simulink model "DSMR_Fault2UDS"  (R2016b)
settings: Solver=FixedStepDiscrete  StartTime=0.0  StopTime=10.0  FixedStep=0.02  RelTol=1e-3  EnableMultiTasking=on
undefined symbols (not defined in the file): bin2dec
libraries: simulink x312
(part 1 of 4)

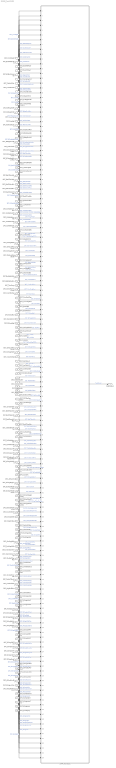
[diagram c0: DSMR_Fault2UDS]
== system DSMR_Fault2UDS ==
  DFC_CurrRngErr : Inport
  DFC_BattVoltRngErr : Inport  Port=2
  DFC_BattHVMsgTmt : Inport  Port=3
  DFC_BusHVMsgTmt : Inport  Port=4
  DFC_638LinCommErr : Inport  Port=5
  DFC_CellTempTmt : Inport  Port=6
  DFC_CellVoltTmt : Inport  Port=7
  DFC_InCanBusOff : Inport  Port=8
  DFC_VeCanBusOff : Inport  Port=9
  DFC_Msg2A3Tmt : Inport  Port=10
  DFC_RcMsg2A3Mis : Inport  Port=11
  DFC_ChkSumMsg2A3Err : Inport  Port=12
  DFC_RcMsg2A5Mis : Inport  Port=13
  DFC_RcMsg2A7Mis : Inport  Port=14
  DFC_CrashNpl : Inport  Port=15
  DFC_FuseNpl : Inport  Port=16
  DFC_Kl30cVoltLoErr : Inport  Port=17
  DFC_PosStuckMax : Inport  Port=18
  DFC_MPosStuckMin : Inport  Port=19
  DFC_MNegStuckMax : Inport  Port=20
  DFC_MNegStuckMin : Inport  Port=21
  DFC_PrStuckMin : Inport  Port=22
  DFC_DChrgPosStuckMax : Inport  Port=23
  DFC_DChrgPosStuckMin : Inport  Port=24
  DFC_DChrgNegStuckMax : Inport  Port=25
  DFC_DChrgNegStuckMin : Inport  Port=26
  DFC_HvPwrUpFail : Inport  Port=27
  DFC_DChrgPwrUpFail : Inport  Port=28
  DFC_BattTAlrmMax : Inport  Port=29
  DFC_BattTFaultMax : Inport  Port=30
  DFC_BattTAlrmMin : Inport  Port=31
  DFC_BattTFaultMin : Inport  Port=32
  DFC_BattTempVldMin : Inport  Port=33
  DFC_BattTCnstMax : Inport  Port=34
  DFC_BattTGradtMax : Inport  Port=35
  DFC_CellVoltAlrmMax : Inport  Port=36
  DFC_CellVoltFaultMax : Inport  Port=37
  DFC_CellVoltFusfMax : Inport  Port=38
  DFC_CellVoltAlrmMin : Inport  Port=39
  DFC_CellVoltFusfMin : Inport  Port=40
  DFC_CellVoltFaultMin : Inport  Port=41
  DFC_CellVoltVldMin : Inport  Port=42
  DFC_CellVoltNpl : Inport  Port=43
  DFC_Msg2E6Tmt : Inport  Port=44
  DFC_RcMsg2E6Mis : Inport  Port=45
  DFC_ChkSumMsg2E6Err : Inport  Port=46
  DFC_RcMsg2E1Mis : Inport  Port=47
  DFC_ChkSumMsg2E1Err : Inport  Port=48
  DFC_DcCanBusOff : Inport  Port=49
  DFC_DChrgTCnntMax : Inport  Port=50
  DFC_ChrgOCNpl : Inport  Port=51
  DFC_DisChOCNpl : Inport  Port=52
  DFC_BattVoltHiMax : Inport  Port=53
  DFC_BattVoltLoMin : Inport  Port=54
  DFC_ThmRnwy : Inport  Port=55
  DFC_AChrgPortOvrTemp : Inport  Port=56
  DFC_CurrOffsPlaus : Inport  Port=57
  DFC_CurrStukPlaus : Inport  Port=58
  DFC_CurrChrgPlaus : Inport  Port=59
  DFC_BattUNpl : Inport  Port=60
  DFC_BattVoltVld : Inport  Port=61
  DFC_PackUNpl : Inport  Port=62
  DFC_PackVoltVld : Inport  Port=63
  DFC_DChrgUNpl : Inport  Port=64
  DFC_DChrgVoltVld : Inport  Port=65
  DFC_BoardTempTmt : Inport  Port=66
  DFC_HvilMax : Inport  Port=67
  DFC_HvilMin : Inport  Port=68
  DFC_HvilSig : Inport  Port=69
  DFC_ChkSumMsg050Err : Inport  Port=70
  DFC_RcMsg050Mis : Inport  Port=71
  DFC_CrashHwNpl : Inport  Port=72
  DFC_IsoChkLv1 : Inport  Port=73
  DFC_IsoChkLv2 : Inport  Port=74
  DFC_InsResValdFault : Inport  Port=75
  DFC_Kl30OutRngErr : Inport  Port=76
  DFC_Kl30VoltLoErr : Inport  Port=77
  DFC_Kl30VoltHiErr : Inport  Port=78
  DFC_EepReadErr : Inport  Port=79
  DFC_BalStuckMax : Inport  Port=80
  DFC_BalStuckMin : Inport  Port=81
  DFC_CSCPwrSpyHiErr : Inport  Port=82
  DFC_CSCPwrSpyLoErr : Inport  Port=83
  DFC_CmcBordOTMax : Inport  Port=84
  DFC_BattTWarnMax : Inport  Port=85
  DFC_BattTWarnMin : Inport  Port=86
  DFC_BattTempVldMax : Inport  Port=87
  DFC_BattTHopMax : Inport  Port=88
  DFC_CellVoltRngHiErr : Inport  Port=89
  DFC_CellVoltRngLoErr : Inport  Port=90
  DFC_CellVoltWarnMax : Inport  Port=91
  DFC_CellVoltWarnMin : Inport  Port=92
  DFC_CellVoltVldMax : Inport  Port=93
  DFC_AChrgCurrMish : Inport  Port=94
  DFC_DChrgCurrMish : Inport  Port=95
  DFC_DChrgLowTempCurrMish : Inport  Port=96
  DFC_AChrgVoltMish : Inport  Port=97
  DFC_DChrgVoltMish : Inport  Port=98
  DFC_DChrgBattTMin : Inport  Port=99
  DFC_CC2Chk : Inport  Port=100
  DFC_APlusChk : Inport  Port=101
  DFC_DChrgMsgTmt : Inport  Port=102
  DFC_DChrgTNegElecMax : Inport  Port=103
  DFC_DChrgTNegElecMin : Inport  Port=104
  DFC_DChrgTNegElecSig : Inport  Port=105
  DFC_DChrgTPosElecMax : Inport  Port=106
  DFC_DChrgTPosElecMin : Inport  Port=107
  DFC_DChrgTPosElecSig : Inport  Port=108
  DFC_CcuSelfChkErr : Inport  Port=109
  DFC_ChrgOCMin : Inport  Port=110
  DFC_ChrgOCMax : Inport  Port=111
  DFC_DisChOCMin : Inport  Port=112
  DFC_DisChOCMax : Inport  Port=113
  DFC_SocRngLoMax : Inport  Port=114
  DFC_SocRngLoMin : Inport  Port=115
  DFC_SocRngHiMax : Inport  Port=116
  DFC_SocRngHiMin : Inport  Port=117
  DFC_InClntOverTmp : Inport  Port=118
  DFC_OutClntOverTmp : Inport  Port=119
  DFC_ClntDsTElecMax : Inport  Port=120
  DFC_ClntDsTElecMin : Inport  Port=121
  DFC_ClntDsTElecSig : Inport  Port=122
  DFC_ClntUsTElecMax : Inport  Port=123
  DFC_ClntUsTElecMin : Inport  Port=124
  DFC_ClntUsTElecSig : Inport  Port=125
  DFC_CoolPerfPlaus : Inport  Port=126
  DFC_HtgPerfPlaus : Inport  Port=127
  DFC_DChrgFobd : Inport  Port=128
  DFC_DChrgHvOnFail : Inport  Port=129
  DFC_AChgHVOnTmt : Inport  Port=130
  DFC_AChgHVOffTmt : Inport  Port=131
  DFC_AChgS2ClsdTmt : Inport  Port=132
  DFC_DChrgStakeErr : Inport  Port=133
  DFC_DChrgStkVoltErr : Inport  Port=134
  DFC_DChrgStkCurrErr : Inport  Port=135
  DFC_AChgPileRdyTmt : Inport  Port=136
  DFC_DChrgCHMTmt : Inport  Port=137
  DFC_DChrgCRMTmt : Inport  Port=138
  DFC_DChrgCMLTmt : Inport  Port=139
  DFC_DChrgCROTmt : Inport  Port=140
  DFC_DChrgCCSTmt : Inport  Port=141
  DFC_DChrgCSTTmt : Inport  Port=142
  DFC_DChrgCSDTmt : Inport  Port=143
  DFC_DChrgParaChk : Inport  Port=144
  DFC_DChrgCableChk : Inport  Port=145
  DFC_DChrgSLACTOut : Inport  Port=146
  DFC_DChrgCnntErr : Inport  Port=147
  DFC_DChrgLckErr : Inport  Port=148
  DFC_AChrgCnntErr : Inport  Port=149
  DFC_AChgLckTmt : Inport  Port=150
  DFC_AChgRdyPndiTmt : Inport  Port=151
  DFC_AChgRdyTmt : Inport  Port=152
  DFC_AChgingErr : Inport  Port=153
  DFC_AChgUnlckTmt : Inport  Port=154
  DFC_AChgFobd : Inport  Port=155
  DFC_SocValJmp : Inport  Port=156
  DSMR_Fault2UDS : Subsystem
  FaultStatus : Outport
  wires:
  DFC_CurrRngErr/1 -> DSMR_Fault2UDS/1(DFC_CurrRngErr)  "DFC_CurrRngErr"
  DFC_BattVoltRngErr/1 -> DSMR_Fault2UDS/2(DFC_BattVoltRngErr)  "DFC_BattVoltRngErr"
  DFC_BattHVMsgTmt/1 -> DSMR_Fault2UDS/3(DFC_BattHVMsgTmt)  "DFC_BattHVMsgTmt"
  DFC_BusHVMsgTmt/1 -> DSMR_Fault2UDS/4(DFC_BusHVMsgTmt)  "DFC_BusHVMsgTmt"
  DFC_638LinCommErr/1 -> DSMR_Fault2UDS/5(DFC_638LinCommErr)  "DFC_638LinCommErr"
  DFC_CellTempTmt/1 -> DSMR_Fault2UDS/6(DFC_CellTempTmt)  "DFC_CellTempTmt"
  DFC_CellVoltTmt/1 -> DSMR_Fault2UDS/7(DFC_CellVoltTmt)  "DFC_CellVoltTmt"
  DFC_InCanBusOff/1 -> DSMR_Fault2UDS/8(DFC_InCanBusOff)  "DFC_InCanBusOff"
  DFC_VeCanBusOff/1 -> DSMR_Fault2UDS/9(DFC_VeCanBusOff)  "DFC_VeCanBusOff"
  DFC_Msg2A3Tmt/1 -> DSMR_Fault2UDS/10(DFC_Msg2A3Tmt)  "DFC_Msg2A3Tmt"
  DFC_RcMsg2A3Mis/1 -> DSMR_Fault2UDS/11(DFC_RcMsg2A3Mis)  "DFC_RcMsg2A3Mis"
  DFC_ChkSumMsg2A3Err/1 -> DSMR_Fault2UDS/12(DFC_ChkSumMsg2A3Err)  "DFC_ChkSumMsg2A3Err"
  DFC_RcMsg2A5Mis/1 -> DSMR_Fault2UDS/13(DFC_RcMsg2A5Mis)  "DFC_RcMsg2A5Mis"
  DFC_RcMsg2A7Mis/1 -> DSMR_Fault2UDS/14(DFC_RcMsg2A7Mis)  "DFC_RcMsg2A7Mis"
  DFC_CrashNpl/1 -> DSMR_Fault2UDS/15(DFC_CrashNpl)  "DFC_CrashNpl"
  DFC_FuseNpl/1 -> DSMR_Fault2UDS/16(DFC_FuseNpl)  "DFC_FuseNpl"
  DFC_Kl30cVoltLoErr/1 -> DSMR_Fault2UDS/17(DFC_Kl30cVoltLoErr)  "DFC_Kl30cVoltLoErr"
  DFC_PosStuckMax/1 -> DSMR_Fault2UDS/18(DFC_PosStuckMax)  "DFC_PosStuckMax"
  DFC_MPosStuckMin/1 -> DSMR_Fault2UDS/19(DFC_MPosStuckMin)  "DFC_MPosStuckMin"
  DFC_MNegStuckMax/1 -> DSMR_Fault2UDS/20(DFC_MNegStuckMax)  "DFC_MNegStuckMax"
  DFC_MNegStuckMin/1 -> DSMR_Fault2UDS/21(DFC_MNegStuckMin)  "DFC_MNegStuckMin"
  DFC_PrStuckMin/1 -> DSMR_Fault2UDS/22(DFC_PrStuckMin)  "DFC_PrStuckMin"
  DFC_DChrgPosStuckMax/1 -> DSMR_Fault2UDS/23(DFC_DChrgPosStuckMax)  "DFC_DChrgPosStuckMax"
  DFC_DChrgPosStuckMin/1 -> DSMR_Fault2UDS/24(DFC_DChrgPosStuckMin)  "DFC_DChrgPosStuckMin"
  DFC_DChrgNegStuckMax/1 -> DSMR_Fault2UDS/25(DFC_DChrgNegStuckMax)  "DFC_DChrgNegStuckMax"
  DFC_DChrgNegStuckMin/1 -> DSMR_Fault2UDS/26(DFC_DChrgNegStuckMin)  "DFC_DChrgNegStuckMin"
  DFC_HvPwrUpFail/1 -> DSMR_Fault2UDS/27(DFC_HvPwrUpFail)  "DFC_HvPwrUpFail"
  DFC_DChrgPwrUpFail/1 -> DSMR_Fault2UDS/28(DFC_DChrgPwrUpFail)  "DFC_DChrgPwrUpFail"
  DFC_BattTAlrmMax/1 -> DSMR_Fault2UDS/29(DFC_BattTAlrmMax)  "DFC_BattTAlrmMax"
  DFC_BattTFaultMax/1 -> DSMR_Fault2UDS/30(DFC_BattTFaultMax)  "DFC_BattTFaultMax"
  DFC_BattTAlrmMin/1 -> DSMR_Fault2UDS/31(DFC_BattTAlrmMin)  "DFC_BattTAlrmMin"
  DFC_BattTFaultMin/1 -> DSMR_Fault2UDS/32(DFC_BattTFaultMin)  "DFC_BattTFaultMin"
  DFC_BattTempVldMin/1 -> DSMR_Fault2UDS/33(DFC_BattTempVldMin)  "DFC_BattTempVldMin"
  DFC_BattTCnstMax/1 -> DSMR_Fault2UDS/34(DFC_BattTCnstMax)  "DFC_BattTCnstMax"
  DFC_BattTGradtMax/1 -> DSMR_Fault2UDS/35(DFC_BattTGradtMax)  "DFC_BattTGradtMax"
  DFC_CellVoltAlrmMax/1 -> DSMR_Fault2UDS/36(DFC_CellVoltAlrmMax)  "DFC_CellVoltAlrmMax"
  DFC_CellVoltFaultMax/1 -> DSMR_Fault2UDS/37(DFC_CellVoltFaultMax)  "DFC_CellVoltFaultMax"
  DFC_CellVoltFusfMax/1 -> DSMR_Fault2UDS/38(DFC_CellVoltFusfMax)  "DFC_CellVoltFusfMax"
  DFC_CellVoltAlrmMin/1 -> DSMR_Fault2UDS/39(DFC_CellVoltAlrmMin)  "DFC_CellVoltAlrmMin"
  DFC_CellVoltFusfMin/1 -> DSMR_Fault2UDS/40(DFC_CellVoltFusfMin)  "DFC_CellVoltFusfMin"
  DFC_CellVoltFaultMin/1 -> DSMR_Fault2UDS/41(DFC_CellVoltFaultMin)  "DFC_CellVoltFaultMin"
  DFC_CellVoltVldMin/1 -> DSMR_Fault2UDS/42(DFC_CellVoltVldMin)  "DFC_CellVoltVldMin"
  DFC_CellVoltNpl/1 -> DSMR_Fault2UDS/43(DFC_CellVoltNpl)  "DFC_CellVoltNpl"
  DFC_Msg2E6Tmt/1 -> DSMR_Fault2UDS/44(DFC_Msg2E6Tmt)  "DFC_Msg2E6Tmt"
  DFC_RcMsg2E6Mis/1 -> DSMR_Fault2UDS/45(DFC_RcMsg2E6Mis)  "DFC_RcMsg2E0Mis"
  DFC_ChkSumMsg2E6Err/1 -> DSMR_Fault2UDS/46(DFC_ChkSumMsg2E6Err)  "DFC_ChkSumMsg2E0Err"
  DFC_RcMsg2E1Mis/1 -> DSMR_Fault2UDS/47(DFC_RcMsg2E1Mis)  "DFC_RcMsg2E1Mis"
  DFC_ChkSumMsg2E1Err/1 -> DSMR_Fault2UDS/48(DFC_ChkSumMsg2E1Err)  "DFC_ChkSumMsg2E1Err"
  DFC_DcCanBusOff/1 -> DSMR_Fault2UDS/49(DFC_DcCanBusOff)  "DFC_DcCanBusOff"
  DFC_DChrgTCnntMax/1 -> DSMR_Fault2UDS/50(DFC_DChrgTCnntMax)  "DFC_DChrgTCnntMax"
  DFC_ChrgOCNpl/1 -> DSMR_Fault2UDS/51(DFC_ChrgOCNpl)  "DFC_ChrgOCNpl"
  DFC_DisChOCNpl/1 -> DSMR_Fault2UDS/52(DFC_DisChOCNpl)  "DFC_DisChOCNpl"
  DFC_BattVoltHiMax/1 -> DSMR_Fault2UDS/53(DFC_BattVoltHiMax)  "DFC_BattVoltHiMax"
  DFC_BattVoltLoMin/1 -> DSMR_Fault2UDS/54(DFC_BattVoltLoMin)  "DFC_BattVoltLoMin"
  DFC_ThmRnwy/1 -> DSMR_Fault2UDS/55(DFC_ThmRnwy)  "DFC_ThmRnwy"
  DFC_AChrgPortOvrTemp/1 -> DSMR_Fault2UDS/56(DFC_AChrgPortOvrTemp)  "DFC_AChrgPortOvrTemp"
  DFC_CurrOffsPlaus/1 -> DSMR_Fault2UDS/57(DFC_CurrOffsPlaus)  "DFC_CurrOffsPlaus"
  DFC_CurrStukPlaus/1 -> DSMR_Fault2UDS/58(DFC_CurrStukPlaus)  "DFC_CurrStukPlaus"
  DFC_CurrChrgPlaus/1 -> DSMR_Fault2UDS/59(DFC_CurrChrgPlaus)  "DFC_CurrChrgPlaus"
  DFC_BattUNpl/1 -> DSMR_Fault2UDS/60(DFC_BattUNpl)  "DFC_BattUNpl"
  DFC_BattVoltVld/1 -> DSMR_Fault2UDS/61(DFC_BattVoltVld)  "DFC_BattVoltVld"
  DFC_PackUNpl/1 -> DSMR_Fault2UDS/62(DFC_PackUNpl)  "DFC_PackUNpl"
  DFC_PackVoltVld/1 -> DSMR_Fault2UDS/63(DFC_PackVoltVld)  "DFC_PackVoltVld"
  DFC_DChrgUNpl/1 -> DSMR_Fault2UDS/64(DFC_DChrgUNpl)  "DFC_DChrgUNpl"
  DFC_DChrgVoltVld/1 -> DSMR_Fault2UDS/65(DFC_DChrgVoltVld)  "DFC_DChrgVoltVld"
  DFC_BoardTempTmt/1 -> DSMR_Fault2UDS/66(DFC_BoardTempTmt)  "DFC_BoardTempTmt"
  DFC_HvilMax/1 -> DSMR_Fault2UDS/67(DFC_HvilMax)  "DFC_HvilMax"
  DFC_HvilMin/1 -> DSMR_Fault2UDS/68(DFC_HvilMin)  "DFC_HvilMin"
  DFC_HvilSig/1 -> DSMR_Fault2UDS/69(DFC_HvilSig)  "DFC_HvilSig"
  DFC_ChkSumMsg050Err/1 -> DSMR_Fault2UDS/70(DFC_ChkSumMsg050Err)  "DFC_ChkSumMsg050Err"
  DFC_RcMsg050Mis/1 -> DSMR_Fault2UDS/71(DFC_RcMsg050Mis)  "DFC_RcMsg050Mis"
  DFC_CrashHwNpl/1 -> DSMR_Fault2UDS/72(DFC_CrashHwNpl)  "DFC_CrashHwNpl"
  DFC_IsoChkLv1/1 -> DSMR_Fault2UDS/73(DFC_IsoChkLv1)  "DFC_IsoChkLv1"
  DFC_IsoChkLv2/1 -> DSMR_Fault2UDS/74(DFC_IsoChkLv2)  "DFC_IsoChkLv2"
  DFC_InsResValdFault/1 -> DSMR_Fault2UDS/75(DFC_InsResValdFault)  "DFC_InsResValdFault"
  DFC_Kl30OutRngErr/1 -> DSMR_Fault2UDS/76(DFC_Kl30OutRngErr)  "DFC_Kl30OutRngErr"
  DFC_Kl30VoltLoErr/1 -> DSMR_Fault2UDS/77(DFC_Kl30VoltLoErr)  "DFC_Kl30VoltLoErr"
  DFC_Kl30VoltHiErr/1 -> DSMR_Fault2UDS/78(DFC_Kl30VoltHiErr)  "DFC_Kl30VoltHiErr"
  DFC_EepReadErr/1 -> DSMR_Fault2UDS/79(DFC_EepReadErr)  "DFC_EepReadErr"
  DFC_BalStuckMax/1 -> DSMR_Fault2UDS/80(DFC_BalStuckMax)  "DFC_BalStuckMax"
  DFC_BalStuckMin/1 -> DSMR_Fault2UDS/81(DFC_BalStuckMin)  "DFC_BalStuckMin"
  DFC_CSCPwrSpyHiErr/1 -> DSMR_Fault2UDS/82(DFC_CSCPwrSpyHiErr)  "DFC_CSCPwrSpyHiErr"
  DFC_CSCPwrSpyLoErr/1 -> DSMR_Fault2UDS/83(DFC_CSCPwrSpyLoErr)  "DFC_CSCPwrSpyLoErr"
  DFC_CmcBordOTMax/1 -> DSMR_Fault2UDS/84(DFC_CmcBordOTMax)  "DFC_CmcBordOTMax"
  DFC_BattTWarnMax/1 -> DSMR_Fault2UDS/85(DFC_BattTWarnMax)  "DFC_BattTWarnMax"
  DFC_BattTWarnMin/1 -> DSMR_Fault2UDS/86(DFC_BattTWarnMin)  "DFC_BattTWarnMin"
  DFC_BattTempVldMax/1 -> DSMR_Fault2UDS/87(DFC_BattTempVldMax)  "DFC_BattTempVldMax"
  DFC_BattTHopMax/1 -> DSMR_Fault2UDS/88(DFC_BattTHopMax)  "DFC_BattTHopMax"
  DFC_CellVoltRngHiErr/1 -> DSMR_Fault2UDS/89(DFC_CellVoltRngHiErr)  "DFC_CellVoltRngHiErr"
  DFC_CellVoltRngLoErr/1 -> DSMR_Fault2UDS/90(DFC_CellVoltRngLoErr)  "DFC_CellVoltRngLoErr"
  DFC_CellVoltWarnMax/1 -> DSMR_Fault2UDS/91(DFC_CellVoltWarnMax)  "DFC_CellVoltWarnMax"
  DFC_CellVoltWarnMin/1 -> DSMR_Fault2UDS/92(DFC_CellVoltWarnMin)  "DFC_CellVoltWarnMin"
  DFC_CellVoltVldMax/1 -> DSMR_Fault2UDS/93(DFC_CellVoltVldMax)  "DFC_CellVoltVldMax"
  DFC_AChrgCurrMish/1 -> DSMR_Fault2UDS/94(DFC_AChrgCurrMish)  "DFC_AChrgCurrMish"
  DFC_DChrgCurrMish/1 -> DSMR_Fault2UDS/95(DFC_DChrgCurrMish)  "DFC_DChrgCurrMish"
  DFC_DChrgLowTempCurrMish/1 -> DSMR_Fault2UDS/96(DFC_DChrgLowTempCurrMish)  "DFC_DChrgLowTempCurrMish"
  DFC_AChrgVoltMish/1 -> DSMR_Fault2UDS/97(DFC_AChrgVoltMish)  "DFC_AChrgVoltMish"
  DFC_DChrgVoltMish/1 -> DSMR_Fault2UDS/98(DFC_DChrgVoltMish)  "DFC_DChrgVoltMish"
  DFC_DChrgBattTMin/1 -> DSMR_Fault2UDS/99(DFC_DChrgBattTMin)  "DFC_DChrgBattTMin"
  DFC_CC2Chk/1 -> DSMR_Fault2UDS/100(DFC_CC2Chk)  "DFC_CC2Chk"
  DFC_APlusChk/1 -> DSMR_Fault2UDS/101(DFC_APlusChk)  "DFC_APlusChk"
  DFC_DChrgMsgTmt/1 -> DSMR_Fault2UDS/102(DFC_DChrgMsgTmt)  "DFC_DChrgMsgTmt"
  DFC_DChrgTNegElecMax/1 -> DSMR_Fault2UDS/103(DFC_DChrgTNegElecMax)  "DFC_DChrgTNegElecMax"
  DFC_DChrgTNegElecMin/1 -> DSMR_Fault2UDS/104(DFC_DChrgTNegElecMin)  "DFC_DChrgTNegElecMin"
  DFC_DChrgTNegElecSig/1 -> DSMR_Fault2UDS/105(DFC_DChrgTNegElecSig)  "DFC_DChrgTNegElecSig"
  DFC_DChrgTPosElecMax/1 -> DSMR_Fault2UDS/106(DFC_DChrgTPosElecMax)  "DFC_DChrgTPosElecMax"
  DFC_DChrgTPosElecMin/1 -> DSMR_Fault2UDS/107(DFC_DChrgTPosElecMin)  "DFC_DChrgTPosElecMin"
  DFC_DChrgTPosElecSig/1 -> DSMR_Fault2UDS/108(DFC_DChrgTPosElecSig)  "DFC_DChrgTPosElecSig"
  DFC_CcuSelfChkErr/1 -> DSMR_Fault2UDS/109(DFC_CcuSelfChkErr)  "DFC_CcuSelfChkErr"
  DFC_ChrgOCMin/1 -> DSMR_Fault2UDS/110(DFC_ChrgOCMin)  "DFC_ChrgOCMin"
  DFC_ChrgOCMax/1 -> DSMR_Fault2UDS/111(DFC_ChrgOCMax)  "DFC_ChrgOCMax"
  DFC_DisChOCMin/1 -> DSMR_Fault2UDS/112(DFC_DisChOCMin)  "DFC_DisChOCMin"
  DFC_DisChOCMax/1 -> DSMR_Fault2UDS/113(DFC_DisChOCMax)  "DFC_DisChOCMax"
  DFC_SocRngLoMax/1 -> DSMR_Fault2UDS/114(DFC_SocRngLoMax)  "DFC_SocRngLoMax"
  DFC_SocRngLoMin/1 -> DSMR_Fault2UDS/115(DFC_SocRngLoMin)  "DFC_SocRngLoMin"
  DFC_SocRngHiMax/1 -> DSMR_Fault2UDS/116(DFC_SocRngHiMax)  "DFC_SocRngHiMax"
  DFC_SocRngHiMin/1 -> DSMR_Fault2UDS/117(DFC_SocRngHiMin)  "DFC_SocRngHiMin"
  DFC_InClntOverTmp/1 -> DSMR_Fault2UDS/118(DFC_InClntOverTmp)  "DFC_InClntOverTmp"
  DFC_OutClntOverTmp/1 -> DSMR_Fault2UDS/119(DFC_OutClntOverTmp)  "DFC_OutClntOverTmp"
  DFC_ClntDsTElecMax/1 -> DSMR_Fault2UDS/120(DFC_ClntDsTElecMax)  "DFC_ClntDsTElecMax"
  DFC_ClntDsTElecMin/1 -> DSMR_Fault2UDS/121(DFC_ClntDsTElecMin)  "DFC_ClntDsTElecMin"
  DFC_ClntDsTElecSig/1 -> DSMR_Fault2UDS/122(DFC_ClntDsTElecSig)  "DFC_ClntDsTElecSig"
  DFC_ClntUsTElecMax/1 -> DSMR_Fault2UDS/123(DFC_ClntUsTElecMax)  "DFC_ClntUsTElecMax"
  DFC_ClntUsTElecMin/1 -> DSMR_Fault2UDS/124(DFC_ClntUsTElecMin)  "DFC_ClntUsTElecMin"
  DFC_ClntUsTElecSig/1 -> DSMR_Fault2UDS/125(DFC_ClntUsTElecSig)  "DFC_ClntUsTElecSig"
  DFC_CoolPerfPlaus/1 -> DSMR_Fault2UDS/126(DFC_CoolPerfPlaus)  "DFC_CoolPerfPlaus"
  DFC_HtgPerfPlaus/1 -> DSMR_Fault2UDS/127(DFC_HtgPerfPlaus)  "DFC_HtgPerfPlaus"
  DFC_DChrgFobd/1 -> DSMR_Fault2UDS/128(DFC_DChrgFobd)  "DFC_DChrgFobd"
  DFC_DChrgHvOnFail/1 -> DSMR_Fault2UDS/129(DFC_DChrgHvOnFail)  "DFC_DChrgHvOnFail"
  DFC_AChgHVOnTmt/1 -> DSMR_Fault2UDS/130(DFC_AChgHVOnTmt)  "DFC_AChgHVOnTmt"
  DFC_AChgHVOffTmt/1 -> DSMR_Fault2UDS/131(DFC_AChgHVOffTmt)  "DFC_AChgHVOffTmt"
  DFC_AChgS2ClsdTmt/1 -> DSMR_Fault2UDS/132(DFC_AChgS2ClsdTmt)  "DFC_AChgS2ClsdTmt"
  DFC_DChrgStakeErr/1 -> DSMR_Fault2UDS/133(DFC_DChrgStakeErr)  "DFC_DChrgStakeErr"
  DFC_DChrgStkVoltErr/1 -> DSMR_Fault2UDS/134(DFC_DChrgStkVoltErr)  "DFC_DChrgStkVoltErr"
  DFC_DChrgStkCurrErr/1 -> DSMR_Fault2UDS/135(DFC_DChrgStkCurrErr)  "DFC_DChrgStkCurrErr"
  DFC_AChgPileRdyTmt/1 -> DSMR_Fault2UDS/136(DFC_AChgPileRdyTmt)  "DFC_AChgPileRdyTmt"
  DFC_DChrgCHMTmt/1 -> DSMR_Fault2UDS/137(DFC_DChrgCHMTmt)  "DFC_DChrgCHMTmt"
  DFC_DChrgCRMTmt/1 -> DSMR_Fault2UDS/138(DFC_DChrgCRMTmt)  "DFC_DChrgCRMTmt"
  DFC_DChrgCMLTmt/1 -> DSMR_Fault2UDS/139(DFC_DChrgCMLTmt)  "DFC_DChrgCMLTmt"
  DFC_DChrgCROTmt/1 -> DSMR_Fault2UDS/140(DFC_DChrgCROTmt)  "DFC_DChrgCROTmt"
  DFC_DChrgCCSTmt/1 -> DSMR_Fault2UDS/141(DFC_DChrgCCSTmt)  "DFC_DChrgCCSTmt"
  DFC_DChrgCSTTmt/1 -> DSMR_Fault2UDS/142(DFC_DChrgCSTTmt)  "DFC_DChrgCSTTmt"
  DFC_DChrgCSDTmt/1 -> DSMR_Fault2UDS/143(DFC_DChrgCSDTmt)  "DFC_DChrgCSDTmt"
  DFC_DChrgParaChk/1 -> DSMR_Fault2UDS/144(DFC_DChrgParaChk)  "DFC_DChrgParaChk"
  DFC_DChrgCableChk/1 -> DSMR_Fault2UDS/145(DFC_DChrgCableChk)  "DFC_DChrgCableChk"
  DFC_DChrgSLACTOut/1 -> DSMR_Fault2UDS/146(DFC_DChrgSLACTOut)  "DFC_DChrgSLACTOut"
  DFC_DChrgCnntErr/1 -> DSMR_Fault2UDS/147(DFC_DChrgCnntErr)  "DFC_DChrgCnntErr"
  DFC_DChrgLckErr/1 -> DSMR_Fault2UDS/148(DFC_DChrgLckErr)  "DFC_DChrgLckErr"
  DFC_AChrgCnntErr/1 -> DSMR_Fault2UDS/149(DFC_AChrgCnntErr)  "DFC_AChrgCnntErr"
  DFC_AChgLckTmt/1 -> DSMR_Fault2UDS/150(DFC_AChgLckTmt)  "DFC_AChgLckTmt"
  DFC_AChgRdyPndiTmt/1 -> DSMR_Fault2UDS/151(DFC_AChgRdyPndiTmt)  "DFC_AChgRdyPndiTmt"
  DFC_AChgRdyTmt/1 -> DSMR_Fault2UDS/152(DFC_AChgRdyTmt)  "DFC_AChgRdyTmt"
  DFC_AChgingErr/1 -> DSMR_Fault2UDS/153(DFC_AChgingErr)  "DFC_AChgingErr"
  DFC_AChgUnlckTmt/1 -> DSMR_Fault2UDS/154(DFC_AChgUnlckTmt)  "DFC_AChgUnlckTmt"
  DFC_AChgFobd/1 -> DSMR_Fault2UDS/155(DFC_AChgFobd)  "DFC_AChgFobd"
  DFC_SocValJmp/1 -> DSMR_Fault2UDS/156(DFC_SocValJmp)  "DFC_SocValJmp"
  DSMR_Fault2UDS/1(FaultStatus) -> FaultStatus/1  "FaultStatus"
